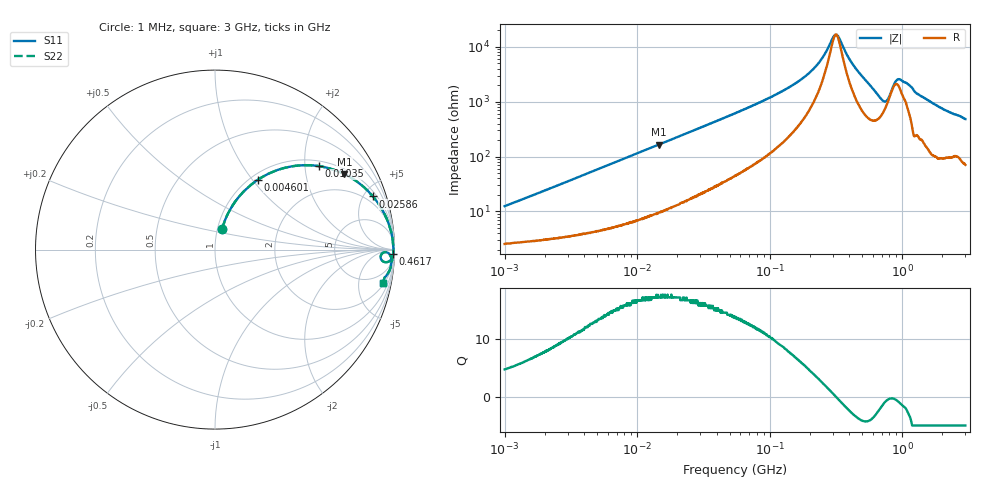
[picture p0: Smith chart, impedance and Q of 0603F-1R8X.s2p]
!s-Parameter Generated by FASTRON Sdn. Bhd.
!FASTRON P/N : 0603F-1R8X
!Keysight Technologies: E4991B_MY54100416_A.01.15
!Date: Wed Jun 19 15:51:18 2024
!Version  :Rev00  Wed Jun 19 15:51:18 2024
!Data & Calibration Information:
!Freq  S11  S21  S12  S22
!PortZ  Port1:50+j0  Port2:50+j0
!When reading reference impedance value at option line is always used.
! Remarks : This data is being provided solely for informational purposes.
# Hz S dB R 50
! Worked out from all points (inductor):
!   1601 points, 1 MHz to 3 GHz, reference 50 ohm
!   read as one part in series: L = 1.92 uH near 1.041 MHz
!   highest Q = 17.4 at 14.54 MHz (marker M1), where L = 1.8 uH
!   self-resonance near 316.8 MHz
!   S11 on the Smith chart (normalised r, x): 1 MHz: 1.05, +0.24; 4.601 MHz: 1.08, +1.07; 10.35 MHz: 1.14, +2.36; 25.86 MHz: 1.35, +5.80; 461.7 MHz: 20, -70; 3 GHz: 2.40, -9.51
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1000000  -18.40 71.4  -0.28 -6.8  -0.28 -6.8  -18.40 71.4
2161090  -12.30 69.1  -0.53 -13.9  -0.53 -13.9  -12.30 69.1
3804036  -8.08 61.9  -1.05 -23.1  -1.05 -23.1  -8.08 61.9
4600725  -6.79 58.4  -1.37 -27.1  -1.37 -27.1  -6.79 58.4
1.034868e7  -2.59 38.8  -4.05 -47.8  -4.05 -47.8  -2.59 38.8
1.447069e7  -1.58 30.4  -5.90 -56.3  -5.90 -56.3  -1.58 30.4
1.454328e7  -1.57 30.3  -5.93 -56.4  -5.93 -56.4  -1.57 30.3
2.585714e7  -0.64 18.6  -9.91 -68.0  -9.91 -68.0  -0.64 18.6
5.504702e7  -0.21 9.1  -16.00 -76.8  -16.00 -76.8  -0.21 9.1
1.269575e8  -0.08 3.5  -24.20 -79.9  -24.20 -79.9  -0.08 3.5
2.083556e8  -0.06 1.5  -31.50 -75.2  -31.50 -75.2  -0.06 1.5
2.457655e8  -0.05 0.9  -35.60 -68.2  -35.60 -68.2  -0.05 0.9
3.002264e8  -0.05 0.2  -43.40 -29.4  -43.40 -29.4  -0.05 0.2
3.172153e8  -0.05 -0.0  -44.60 0.8  -44.60 0.8  -0.05 -0.0
4.616833e8  -0.06 -1.5  -31.30 73.4  -31.30 73.4  -0.06 -1.5
7.028992e8  -0.44 -4.2  -21.20 53.5  -21.20 53.5  -0.44 -4.2
7.50144e8  -0.66 -3.3  -20.70 35.4  -20.70 35.4  -0.66 -3.3
7.925923e8  -0.65 -1.6  -22.20 20.1  -22.20 20.1  -0.65 -1.6
8.892696e8  -0.33 -1.0  -27.60 24.3  -27.60 24.3  -0.33 -1.0
9.585869e8  -0.23 -1.6  -28.40 45.3  -28.40 45.3  -0.23 -1.6
1.704314e9  -0.15 -6.0  -19.60 77.6  -19.60 77.6  -0.15 -6.0
3e9  -0.43 -11.3  -14.10 70.3  -14.10 70.3  -0.43 -11.3
